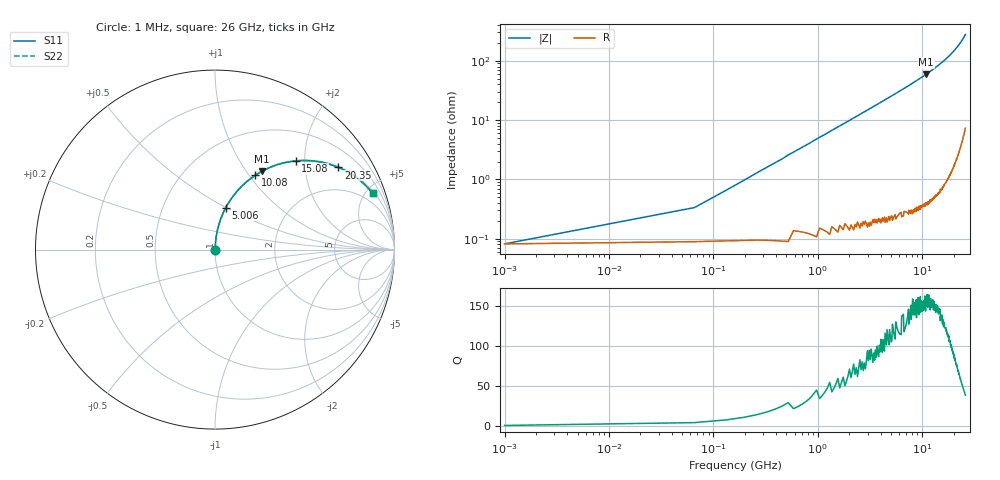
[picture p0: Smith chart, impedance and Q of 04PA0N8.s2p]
! Coilcraft 0402PA-0N8 Chip Inductor
! 11 March 2004
# MHZ S MA R 50
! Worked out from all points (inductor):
!   401 points, 1 MHz to 26 GHz, reference 50 ohm
!   read as one part in series: L = 781 pH near 131 MHz
!   highest Q = 156 at 10.92 GHz (marker M1), where L = 863 pH
!   S11 on the Smith chart (normalised r, x): 1 MHz: 1.00, +0.00; 5.006 GHz: 1.00, +0.50; 10.08 GHz: 1.01, +1.07; 15.08 GHz: 1.01, +1.81; 20.35 GHz: 1.04, +2.98; 26 GHz: 1.15, +5.55
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1  0.0006359 4.4  0.999 -0.0  0.999 -0.0  0.0006359 4.4
65.998  0.003327 76.1  0.999 -0.2  0.999 -0.2  0.003327 76.1
195.992  0.00964 84.0  0.999 -0.6  0.999 -0.6  0.00964 84.0
260.99  0.013 85.0  0.999 -0.7  0.999 -0.7  0.013 85.0
390.985  0.019 85.8  0.999 -1.1  0.999 -1.1  0.019 85.8
520.98  0.026 86.0  0.999 -1.5  0.999 -1.5  0.026 86.0
650.975  0.032 86.1  0.998 -1.8  0.998 -1.8  0.032 86.1
910.965  0.045 85.8  0.998 -2.6  0.998 -2.6  0.045 85.8
1430.945  0.07 84.8  0.996 -4.0  0.996 -4.0  0.07 84.8
2210.915  0.108 82.9  0.993 -6.2  0.993 -6.2  0.108 82.9
3250.875  0.158 80.2  0.986 -9.1  0.986 -9.1  0.158 80.2
4355.832  0.211 77.2  0.975 -12.2  0.975 -12.2  0.211 77.2
5005.808  0.242 75.5  0.968 -14.0  0.968 -14.0  0.242 75.5
8710.665  0.413 65.2  0.908 -24.4  0.908 -24.4  0.413 65.2
10075.61  0.472 61.5  0.878 -28.2  0.878 -28.2  0.472 61.5
10920.58  0.508 59.1  0.858 -30.5  0.858 -30.5  0.508 59.1
13000.5  0.591 53.4  0.803 -36.2  0.803 -36.2  0.591 53.4
15080.42  0.668 47.7  0.739 -41.9  0.739 -41.9  0.668 47.7
17355.33  0.743 41.5  0.663 -48.0  0.663 -48.0  0.743 41.5
20345.22  0.826 33.6  0.554 -55.7  0.554 -55.7  0.826 33.6
21710.17  0.858 30.1  0.502 -59.1  0.502 -59.1  0.858 30.1
26000  0.933 19.6  0.336 -68.9  0.336 -68.9  0.933 19.6
